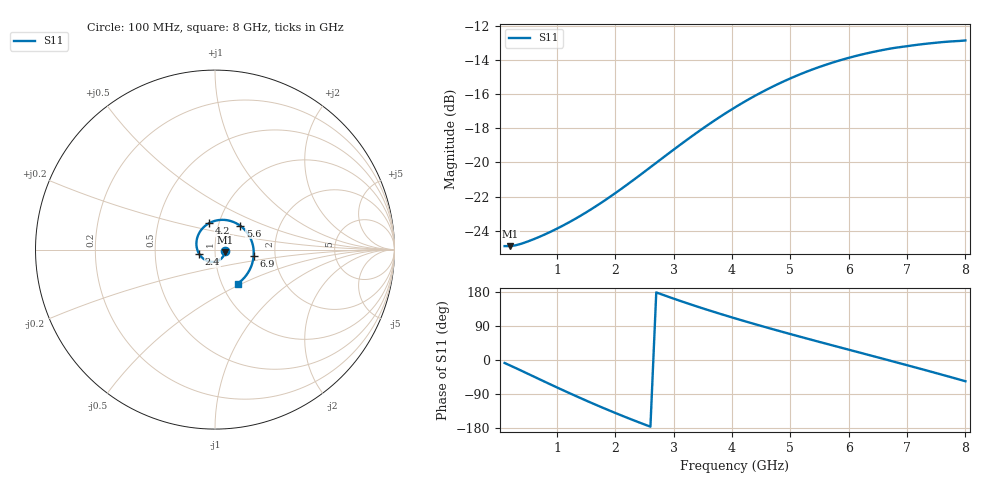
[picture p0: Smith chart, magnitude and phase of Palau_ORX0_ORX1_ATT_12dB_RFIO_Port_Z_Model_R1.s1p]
! Created Fri Oct  9 14:28:18 2020
! Palau ORX0/ORX1 RFIO Port Impedance Model.
! Attenuation  : 12 dB.
! Revision		: R1.
! Impedance Mode 	: Balanced Differential-Mode.
! Impedance Format 	: Series Equivalent Differential Impedance (SEDZ).
# hz S ma R 100
! 1 Port Network Data from SP1.SP block
! freq  magS11  angS11
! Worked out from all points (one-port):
!   80 points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, 100 MHz to 8 GHz, reference 100 ohm
!   lowest |S11| = -24.9 dB at 200 MHz (marker M1), VSWR 1.12, Z = 112 - j3.26 ohm
!   |S11| at or under -10 dB: start of sweep to end of sweep
!   S11 on the Smith chart (normalised r, x): 100 MHz: 1.12, -0.02; 2.4 GHz: 0.84, -0.04; 4.2 GHz: 0.90, +0.27; 5.6 GHz: 1.27, +0.35; 6.9 GHz: 1.54, -0.12; 8 GHz: 1.19, -0.47
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1e8  0.05686 -7.9
2e8  0.05684 -14.9
6e8  0.05959 -43.7
1.1e9  0.06531 -79.6
1.4e9  0.06976 -100.4
1.6e9  0.07321 -113.9
1.8e9  0.07706 -127.1
2.1e9  0.08367 -146.1
2.4e9  0.09127 -164.3
2.8e9  0.1028 172.7
3.1e9  0.1124 156.6
3.3e9  0.119 146.2
3.6e9  0.1293 131.3
4.1e9  0.1468 107.7
4.2e9  0.1503 103.2
4.5e9  0.1605 89.9
4.7e9  0.167 81.2
5.1e9  0.1795 64.2
5.3e9  0.1852 55.9
5.6e9  0.1932 43.6
5.8e9  0.1982 35.4
6.1e9  0.2048 23.2
6.5e9  0.2123 6.8
6.9e9  0.2181 -9.6
7.1e9  0.2205 -17.8
7.5e9  0.2245 -34.6
7.7e9  0.2261 -43.1
8e9  0.2279 -56.0
